// TwinCAT 3 PLC project NCI_sample
// ProgramVersion: 3.1.4022.1
// libraries:
//   Tc2_MC2, * (Beckhoff Automation GmbH)
//   Tc2_NCI, * (Beckhoff Automation GmbH)
//   Tc2_PlcInterpolation, * (Beckhoff Automation GmbH)
//   Tc2_Standard, * (Beckhoff Automation GmbH)
//   Tc2_System, * (Beckhoff Automation GmbH)
//   Tc3_Module, * (Beckhoff Automation GmbH)
// project tree:
//   / PlcTask.TcTTO
//   POUs/ FB_EnableAxes.TcPOU, FB_SimpleNciSequence.TcPOU, MAIN.TcPOU
// real-time tasks:
//   TASK PlcTask: cycle T#10ms, priority 20, ADS port 350
// motion (NC):
//   TASK NC-Task 1 SAF: cycle T#2ms, priority 4, ADS port 501
//   TASK NC-Task 1 SVB: cycle T#10ms, priority 8, ADS port 511
//   AXIS X (id 1)
//     OtherSettings: AllowMotionCmdToSlave=true
//     encoder EncType=1
//     drive DrvType=5
//       Analog: ScaleFactorActTorque=0.1
//     controller CtrType=1
//       CtrPara: PriorControlFactor=1
//         Observer: BandWidth=20
//   AXIS Y (id 2)
//     OtherSettings: AllowMotionCmdToSlave=true
//     encoder EncType=1
//     drive DrvType=5
//       Analog: ScaleFactorActTorque=0.1
//     controller CtrType=1
//       CtrPara: PriorControlFactor=1
//         Observer: BandWidth=20
//   AXIS Z (id 3)
//     OtherSettings: AllowMotionCmdToSlave=true
//     encoder EncType=1
//     drive DrvType=5
//       Analog: ScaleFactorActTorque=0.1
//     controller CtrType=1
//       CtrPara: PriorControlFactor=1
//         Observer: BandWidth=20
//   AXIS Q1 (id 4)
//     OtherSettings: AllowMotionCmdToSlave=true
//     encoder EncType=1
//     drive DrvType=5
//       Analog: ScaleFactorActTorque=0.1
//     controller CtrType=1
//       CtrPara: PriorControlFactor=1
//         Observer: BandWidth=20
//   AXIS Q2 (id 5)
//     OtherSettings: AllowMotionCmdToSlave=true
//     encoder EncType=1
//     drive DrvType=5
//       Analog: ScaleFactorActTorque=0.1
//     controller CtrType=1
//       CtrPara: PriorControlFactor=1
//         Observer: BandWidth=20
//   AXIS Q3 (id 6)
//     OtherSettings: AllowMotionCmdToSlave=true
//     encoder EncType=1
//     drive DrvType=5
//       Analog: ScaleFactorActTorque=0.1
//     controller CtrType=1
//       CtrPara: PriorControlFactor=1
//         Observer: BandWidth=20
// variable links:
//   NCI_sample/NCI_sample Instance <-> NC-Task 1 SAF/Axes/Q1
//     PlcTask Inputs/MAIN.io_Q1.NcToPlc <-> Outputs/ToPlc
//     PlcTask Outputs/MAIN.io_Q1.PlcToNc <-> Inputs/FromPlc
//   NCI_sample/NCI_sample Instance <-> NC-Task 1 SAF/Axes/Q2
//     PlcTask Inputs/MAIN.io_Q2.NcToPlc <-> Outputs/ToPlc
//     PlcTask Outputs/MAIN.io_Q2.PlcToNc <-> Inputs/FromPlc
//   NCI_sample/NCI_sample Instance <-> NC-Task 1 SAF/Axes/Q3
//     PlcTask Inputs/MAIN.io_Q3.NcToPlc <-> Outputs/ToPlc
//     PlcTask Outputs/MAIN.io_Q3.PlcToNc <-> Inputs/FromPlc
//   NCI_sample/NCI_sample Instance <-> NC-Task 1 SAF/Axes/X
//     PlcTask Inputs/MAIN.io_X.NcToPlc <-> Outputs/ToPlc
//     PlcTask Outputs/MAIN.io_X.PlcToNc <-> Inputs/FromPlc
//   NCI_sample/NCI_sample Instance <-> NC-Task 1 SAF/Axes/Y
//     PlcTask Inputs/MAIN.io_Y.NcToPlc <-> Outputs/ToPlc
//     PlcTask Outputs/MAIN.io_Y.PlcToNc <-> Inputs/FromPlc
//   NCI_sample/NCI_sample Instance <-> NC-Task 1 SAF/Axes/Z
//     PlcTask Inputs/MAIN.io_Z.NcToPlc <-> Outputs/ToPlc
//     PlcTask Outputs/MAIN.io_Z.PlcToNc <-> Inputs/FromPlc
//   NCI_sample/NCI_sample Instance <-> NC-Task 1 SAF/Channel 2
//     PlcTask Inputs/MAIN.in_stItpToPlc <-> Outputs/ToPlc
//     PlcTask Outputs/MAIN.out_stPlcToItp <-> Inputs/FromPlc

CONFIGURATION NCI_sample
    RESOURCE PLC ON TwinCAT3
        TASK PlcTask(INTERVAL := T#10ms, PRIORITY := 20);
        PROGRAM MAIN WITH PlcTask : MAIN;
    END_RESOURCE
END_CONFIGURATION

// ---- POUs/MAIN.TcPOU
PROGRAM MAIN
VAR
	bUserEnableAxes:		BOOL	:= TRUE;		(*触发使能功能块，由于是模拟程序，所以直接对轴租进行使能*)
	fUserOverride:			LREAL	:= 100.0;		(*设置通道速比为100%*)
	
	io_X:					AXIS_REF;				(*定义各NC轴*)
	io_Y:					AXIS_REF;
	io_Z:					AXIS_REF;
	io_Q1:					AXIS_REF;
	io_Q2:					AXIS_REF;
	io_Q3:					AXIS_REF;
	
	in_stItpToPlc	AT %I*:	NcToPlc_NciChannel_Ref;	(*定义NCI通道反馈给PLC的一系列状态字等*)
	out_stPlcToItp	AT %Q*:	PLCTONC_NCICHANNEL_REF; (*定义PLC发送给NCI通道的一系列状控制字等*)

	fbEnableAxes:			FB_EnableAxes;			(*调用轴组使能功能块*)
	bAllAxesReady:			BOOL;					(*该变量用于标明轴组使能成功*)
	
	
	fbSimpleNciSequence:	FB_SimpleNciSequence;	(*调用生成NCI通道及执行G代码的功能块*)
	bExecSimpleNci:			BOOL	:= FALSE;		(*用于触发生成NCI通道及执行G代码的功能块*)
	bExeConfirmHsk: 		BOOL	:= FALSE;		(*用于确认M握手指令*)
	sPrgName:				STRING(255) :='Gtest.nc';	(*放置在安装盘中TwinCAT\MC\NCI的文件夹*)
END_VAR

//==========================================
// NciSimpleSample V1.1
//==========================================

//==========================================
// This sample should illustrate how to start up an NCI project.
// Error handling is missing and the sample is not commplete to run a machine.
// 
// To run program copy G-Code file (first.nc) 
// to folder 'C:\TwinCAT\Mc\Nci'.
// Then set bExecSimpleNci to TRUE.
//==========================================
fbEnableAxes(
	bEnableAxes:= bUserEnableAxes, 
	stX:=io_X , 
	stY:=io_Y , 
	stZ:=io_Z , 
	stM1:=io_Q1 , 
	stM2:=io_Q2 , 
	stM3:=io_Q3 , 
	bAllAxesReady=>bAllAxesReady );
	
ItpSetOverridePercent(fOverridePercent:=fUserOverride , sPlcToNci:=out_stPlcToItp);

fbSimpleNciSequence(
	bExecute:=bExecSimpleNci , 
	bConfirmHsk:=bExeConfirmHsk , 
	sPrgName:=sPrgName , 
	bBusy=> , 
	bError=> , 
	bDone=> , 
	stX:=io_X , 
	stY:= io_Y, 
	stZ:= io_Z, 
	st_Q1:=io_Q1 , 
	st_Q2:=io_Q2 , 
	st_Q3:= io_Q3, 
	stItpToPlc:=in_stItpToPlc, 
	stPlcToItp:= out_stPlcToItp);

END_PROGRAM

// ---- POUs/FB_EnableAxes.TcPOU
FUNCTION_BLOCK FB_EnableAxes
VAR_INPUT
	bEnableAxes: BOOL:= TRUE;
END_VAR
VAR_OUTPUT
	bAllAxesReady:	BOOL:= FALSE;
END_VAR
VAR_IN_OUT
	stX:	AXIS_REF;
	stY:	AXIS_REF;
	stZ:	AXIS_REF;
	stM1:	AXIS_REF;
	stM2:	AXIS_REF;
	stM3:	AXIS_REF;
END_VAR
VAR
	fOverride:	LREAL	:= 100.0;
	fbPowerX:	MC_Power;
	fbPowerY:	MC_Power;
	fbPowerZ:	MC_Power;
	fbPowerM1:	MC_Power;
	fbPowerM2:	MC_Power;
	fbPowerM3:	MC_Power;
END_VAR

stX.ReadStatus();
stY.ReadStatus();
stZ.ReadStatus();
stM1.ReadStatus();
stM2.ReadStatus();
stM3.ReadStatus();


fbPowerX(
	Enable:=bEnableAxes, 
	Enable_Positive:=bEnableAxes, 
	Enable_Negative:=bEnableAxes, 
	Override:=fOverride, 
	BufferMode:= , 
	Axis:=stX, 
	Status=> , 
	Busy=> , 
	Active=> , 
	Error=> , 
	ErrorID=> );
fbPowerY(
	Enable:=bEnableAxes, 
	Enable_Positive:=bEnableAxes, 
	Enable_Negative:=bEnableAxes, 
	Override:=fOverride, 
	BufferMode:= , 
	Axis:=stY, 
	Status=> , 
	Busy=> , 
	Active=> , 
	Error=> , 
	ErrorID=> );	
fbPowerZ(
	Enable:=bEnableAxes, 
	Enable_Positive:=bEnableAxes, 
	Enable_Negative:=bEnableAxes, 
	Override:=fOverride, 
	BufferMode:= , 
	Axis:=stZ, 
	Status=> , 
	Busy=> , 
	Active=> , 
	Error=> , 
	ErrorID=> );	
fbPowerM1(
	Enable:=bEnableAxes, 
	Enable_Positive:=bEnableAxes, 
	Enable_Negative:=bEnableAxes, 
	Override:=fOverride, 
	BufferMode:= , 
	Axis:=stM1, 
	Status=> , 
	Busy=> , 
	Active=> , 
	Error=> , 
	ErrorID=> );	
fbPowerM2(
	Enable:=bEnableAxes, 
	Enable_Positive:=bEnableAxes, 
	Enable_Negative:=bEnableAxes, 
	Override:=fOverride, 
	BufferMode:= , 
	Axis:=stM2, 
	Status=> , 
	Busy=> , 
	Active=> , 
	Error=> , 
	ErrorID=> );	
fbPowerM3(
	Enable:=bEnableAxes, 
	Enable_Positive:=bEnableAxes, 
	Enable_Negative:=bEnableAxes, 
	Override:=fOverride, 
	BufferMode:= , 
	Axis:=stM3, 
	Status=> , 
	Busy=> , 
	Active=> , 
	Error=> , 
	ErrorID=> );	
bAllAxesReady	:= fbPowerX.Status AND fbPowerY.Status AND fbPowerZ.Status AND 
	fbPowerM1.Status AND fbPowerM2.Status AND fbPowerM3.Status;

END_FUNCTION_BLOCK

// ---- POUs/FB_SimpleNciSequence.TcPOU
FUNCTION_BLOCK FB_SimpleNciSequence
VAR_INPUT
	bExecute			: BOOL;						(*触发位*)
	bConfirmHsk			: BOOL	:= FALSE;			(*确认H握手代码*)
	sPrgName			: STRING(255) ;				(*G代码所在地址*)
END_VAR
VAR_OUTPUT
	bBusy				: BOOL;						(*功能块在被执行*)
	bError				: BOOL;						(*出现报错*)
	bDone				: BOOL;						(*功能块被执行完毕*)
END_VAR
VAR_IN_OUT
	stX					: AXIS_REF;					(*通道的X轴*)
	stY					: AXIS_REF;					(*通道的Y轴*)
	stZ					: AXIS_REF;					(*通道的Z轴*)
	st_Q1				: AXIS_REF;					(*通道的辅助Q1轴*)
	st_Q2				: AXIS_REF;					(*通道的辅助Q2轴*)
	st_Q3				: AXIS_REF;					(*通道的辅助Q3轴*) 
	stItpToPlc			: NCTOPLC_NCICHANNEL_REF;	(*NCI通道反馈给PLC的*)
	stPlcToItp			: PLCTONC_NCICHANNEL_REF;	(*PLC发送给NCI通道的*)
END_VAR
VAR
	nState				: UDINT	:= 0;				
	nErrorState			: UDINT;
	
	fbBuildGroup		: CfgBuildExt3DGroup;		(*创建通道，并将轴添加进通道*)
	fbLoadGCode			: ItpLoadProgEx;			(*装载G代码*)
	fbStartGCode		: ItpStartStopEx;			(*开始执行G代码*)
	fbClearGroup		: CfgReconfigGroup;			(*清除NCI通道中的周，释放轴*)
	fbConfirmHsk		: ItpConfirmHsk;			(*确认H握手代码*)
	
	nInterpreterState	: UDINT	:= 0;
	
	
END_VAR

CASE nState OF
0:
	IF bExecute THEN			(*功能块的触发位一旦触发后，执行以下：*)
		bBusy	:= TRUE;		(*FB为执行状态*)
		bDone	:= FALSE;		(*对执行完毕功能快的引脚复位*)
		bError	:= FALSE;		(*报错引脚复位*)
		nErrorState	:= nState;	(*nstate为0，认为无报错*)
		nState	:= 10;			(*进入10步*)
	END_IF	
	
10:
	// 该步用来将NC轴添加进NCI通道中
	fbBuildGroup(
		bExecute:=TRUE, 
		nGroupId:=ItpGetGroupId(sNciToPlc:=stItpToPlc) , 
		nXAxisId:=stX.NcToPlc.AxisId, 
		nYAxisId:=stY.NcToPlc.AxisId, 
		nZAxisId:=stZ.NcToPlc.AxisId, 
		nQ1AxisId:=st_Q1.NcToPlc.AxisId, 
		nQ2AxisId:=st_Q2.NcToPlc.AxisId, 
		nQ3AxisId:=st_Q3.NcToPlc.AxisId, 
		nQ4AxisId:= 0, 
		nQ5AxisId:= 0, 
		tTimeOut:= , 
		bBusy=> , 
		bErr=> , 
		nErrId=> );
	IF NOT fbBuildGroup.bBusy THEN
		IF NOT fbBuildGroup.bErr THEN
			nState	:= 20;(*如果将NC轴添加进NCI通道中成功后，进入20步*)
		ELSE
			(* add error handling *)
			nErrorState	:= nState;(*如果出现报错，首先FB出现报错，然后将错误状态定位在10步，并且进入9999步*)
			bBusy	:= FALSE;
			bError	:= TRUE;
			nState	:= 9999;
		END_IF
		fbBuildGroup(bExecute:=FALSE); (*对fbBuildGroup的触发位复位*)
	END_IF
	
20:
	(*将G代码装在进通道，sPrgName有两种用法，第一种写出路径+G代码程序的文件名，第二种直接写G代码程序的文件名,但需要放置在安装盘中TwinCAT\MC\NCI的文件夹*)
	// load g-code file 
	// pls. ensure that first.nc is available in TwinCAT\MC\NCI-folder 
	fbLoadGCode(
		sNciToPlc:=stItpToPlc, 
		bExecute:=TRUE, 
		sPrg:= sPrgName, 
		nLength:= INT_TO_UDINT(LEN(sPrgName)), 
		tTimeOut:= , 
		bBusy=> , 
		bErr=> , 
		nErrId=> );
	IF NOT fbLoadGCode.bBusy THEN
		IF NOT fbLoadGCode.bErr THEN
			nState	:= 30;(*如果装载G代码成功后，进入20步*)
		ELSE
			(* add error handling *)
			nErrorState	:= nState;(*如果出现报错，首先FB出现报错，然后将错误状态定位在20步，并且进入9999步*)
			bBusy	:= FALSE;
			bError	:= TRUE;
			nState	:= 9999;				
		END_IF
		fbLoadGCode(sNciToPlc:=stItpToPlc, bExecute:=FALSE); (*对fbLoadGCode的触发位复位*)
	END_IF
	
30:
	(*检查通道状态，如果处于ready，那么说明装载G代码成功*)
	// we have to check the status of the interpreter. It has to be in ready state, in case of loading the program successfully.
	nInterpreterState	:= ItpGetStateInterpreter(sNciToPlc:=stItpToPlc);(*获取通道当前状态*)
	IF nInterpreterState = Tc2_NCI.NCI_INTERPRETER_READY THEN(*判断通道是否为ready状态*)
		nState	:= 40;
	ELSE
		(* add error handling *)
		nErrorState	:= nState;(*如果通道没有到ready状态，将错误状态定位在30步，并且进入9999步*)
		bBusy	:= FALSE;
		bError	:= TRUE;
		nState	:= 9999;				
	END_IF
	
40:
	(*开始执行G代码*)
	// start g-code file
	fbStartGCode(
		bStart:=TRUE, 
		bStop:=FALSE, 
		tTimeOut:= , 
		sNciToPlc:= stItpToPlc, 
		bBusy=> , 
		bErr=> , 
		nErrId=> );
	IF NOT fbStartGCode.bBusy THEN
		IF NOT fbStartGCode.bErr THEN(*如果开始执行G代码了，进入50步*)
			nState	:= 50;
		ELSE	
			(* add error handling *)
			nErrorState	:= nState;(*如果未能成功执行，将错误状态定位在40步，并且进入9999步*)
			bBusy	:= FALSE;
			bError	:= TRUE;
			nState	:= 9999;				
		END_IF
		fbStartGCode( bStart:=FALSE, sNciToPlc:= stItpToPlc ); (*对fbStartGCode的触发位复位*)
	END_IF
	
50:
	(*检查状态，确认G代码是否执行完毕*)
	// check state, again - we are at least not in ready state for several ticks
	// this is to ensure that we don't indicate program has finished, before we have started 
	nInterpreterState	:= ItpGetStateInterpreter(sNciToPlc:=stItpToPlc);
	IF nInterpreterState <> Tc2_NCI.NCI_INTERPRETER_READY THEN(*判断通道是否为ready状态*)
		// nci is running
		nState	:= 60;(*不为ready的状态，进入60步*)
	END_IF

60:
	(*获取通道的当前状态*)
	nInterpreterState	:= ItpGetStateInterpreter(sNciToPlc:=stItpToPlc);
	IF	nInterpreterState = Tc2_NCI.NCI_INTERPRETER_READY THEN(*判断是否回到ready状态，回到说明G代码已经执行完毕,进入70步*)
		// program has finished
		nState	:= 70;
	ELSIF nInterpreterState = Tc2_NCI.NCI_INTERPRETER_ABORTED THEN(*如果通道状态变成aborted的话，说明通道此时出现报错，具体需要通过通道报错的ID进行排查原因*)
		// a run-time error occured - this could be a lag error or something else... 
		// add error handling
		;
	END_IF	
70:
	(*G代码执行完毕，释放NC轴，解散NCI通道*)
	// program has finished 
	// now clear interpolation group 
	fbClearGroup(
		bExecute:=TRUE, 
		nGroupId:=ItpGetGroupId(sNciToPlc:=stItpToPlc) , 
		tTimeOut:= , 
		bBusy=> , 
		bErr=> , 
		nErrId=> );
	IF NOT fbClearGroup.bBusy THEN
		IF NOT fbClearGroup.bErr THEN(*如果释放完毕，进入80步*)
			nState	:= 80;
		ELSE
			(* add error handling *)
			nErrorState	:= nState;(*如果未能成功执行，将错误状态定位在70步，并且进入9999步*)
			bBusy	:= FALSE;
			bError	:= TRUE;
			nState	:= 9999;				
		END_IF
		fbClearGroup(bExecute:=FALSE); (*对fbClearGroup的触发位复位*)
	END_IF
80:
	(*以上已经完成该功能块的目标，对输出位DONE置为TRUE，说明已完成G代码的执行*)
	bDone	:= TRUE;
	bBusy	:= FALSE;
	IF NOT bExecute THEN(*若此功能块的触发位没有复位，那么nState回到0步*)
		nState	:= 0;
	END_IF
9999:
	// error state 
	IF NOT bExecute THEN(*若此功能块的触发位没有复位,那么回到初始0步，重新执行*)
		nState	:= 0;
		bError	:= FALSE;
	END_IF
END_CASE

// handling of m-functions is done outside statemachine
// all m-functions are directly confiremd. In a real application we have of course to consider the m-function numbers to turn on/off certain functions in the machine.
(*原程序部分对H握手型直接做了复位，将此部分屏蔽，保留确认功能块
IF ItpIsHskMFunc(stItpToPlc) AND NOT fbConfirmHsk.bBusy THEN
	bConfirmHsk	:= TRUE;
ELSE	
	bConfirmHsk	:= FALSE;
END_IF	
*)

(*一旦G代码中出现M握手型，用于进行确认M握手指令*)
fbConfirmHsk(
	bExecute:=bConfirmHsk , 
	sNciToPlc:=stItpToPlc , 
	sPlcToNci:=stPlcToItp , 
	bBusy=> , 
	bErr=> , 
	nErrId=> );

END_FUNCTION_BLOCK
